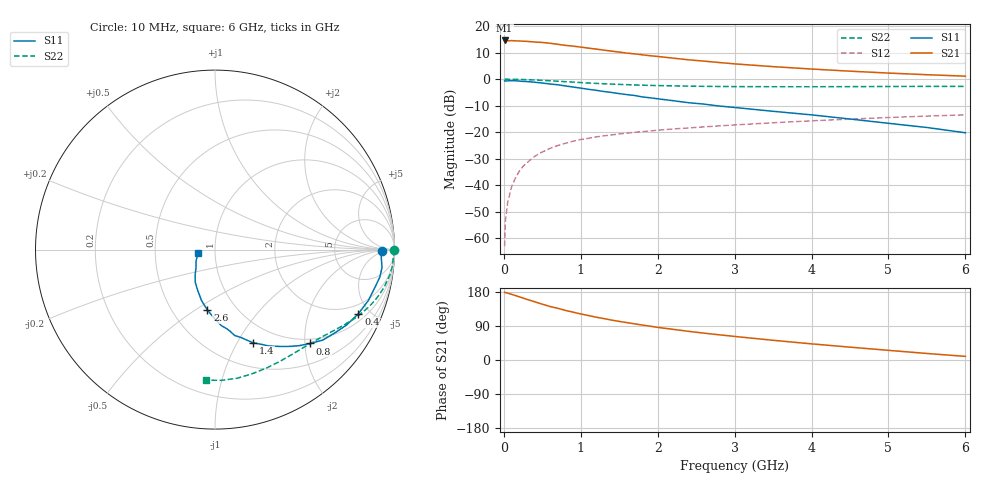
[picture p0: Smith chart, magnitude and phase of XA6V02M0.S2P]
! SIEMENS Discrete & RF Semiconductors
! BFY180
! Si NPN RF Bipolar Junction Transistor in MICRO-X
! VCE = 6 V  IC = 2 mA
! Common Emitter S-Parameters:  May  1997
# GHz  S  MA  R  50
!  f  S11  S21  S12  S22
! GHz  MAG  ANG  MAG  ANG  MAG  ANG  MAG  ANG
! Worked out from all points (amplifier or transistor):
!   36 points, 10 MHz to 6 GHz, reference 50 ohm
!   highest |S21| = 14.6 dB at 10 MHz (marker M1)
!   |S21| within 3 dB of that: start of sweep to 1.127 GHz
!   unconditionally stable (mu >= 1): 3.067 GHz to end of sweep
!   at 250 MHz: K = 0.12, MSG = 23.6 dB, |S12| = -32.9 dB
!   at 1.4 GHz: K = 0.64, MSG = 15.8 dB, |S12| = -21.1 dB
!   at 6 GHz: K = 1.06, MAG = 5.8 dB, |S12| = -13.5 dB
!   S11 on the Smith chart (normalised r, x): 10 MHz: 27, -3; 400 MHz: 1.39, -4.25; 800 MHz: 0.90, -2.12; 1.4 GHz: 0.77, -1.17; 2.6 GHz: 0.74, -0.56; 6 GHz: 0.83, -0.04
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0.01  0.9302 -0.4  5.383 178.7  0.0007 82.9  0.9952 -0.2
0.02  0.9262 -1.1  5.382 178.0  0.0021 99.5  0.9999 -0.6
0.05  0.928 -3.1  5.292 176.5  0.0047 88.1  0.9955 -1.6
0.1  0.936 -6.1  5.353 173.4  0.0092 84.8  0.9933 -3.3
0.25  0.9081 -15.5  5.211 163.6  0.0226 80.6  0.9846 -8.1
0.3  0.9006 -18.3  5.173 160.0  0.0263 78.6  0.9779 -9.6
0.4  0.8751 -24.1  5.03 153.7  0.0348 74.6  0.9654 -12.5
0.5  0.8446 -29.9  4.936 147.3  0.0421 71.2  0.9491 -15.4
0.6  0.8107 -35.2  4.767 141.1  0.0492 68.4  0.9321 -18.0
0.8  0.745 -44.6  4.345 130.9  0.0614 62.9  0.8956 -22.7
1  0.6766 -52.9  4.034 121.5  0.0724 57.8  0.8627 -26.8
1.1  0.643 -57.0  3.853 117.3  0.0764 55.9  0.8462 -28.5
1.4  0.5606 -67.8  3.384 105.4  0.0883 51.3  0.806 -33.6
1.5  0.5339 -70.7  3.246 101.8  0.0922 49.8  0.7957 -35.0
1.8  0.4619 -79.6  2.881 92.2  0.1023 46.7  0.7693 -39.2
2  0.4259 -85.1  2.682 86.1  0.1085 44.7  0.7565 -41.8
2.2  0.392 -89.4  2.495 80.9  0.1146 42.8  0.7475 -44.6
2.6  0.3381 -97.2  2.192 70.9  0.1255 39.9  0.732 -49.5
3.5  0.2472 -112.9  1.724 52.0  0.1501 33.7  0.7197 -60.5
4.5  0.1766 -128.7  1.415 33.9  0.1758 26.7  0.7223 -73.3
5.5  0.1221 -149.5  1.213 17.2  0.2007 19.0  0.7294 -87.0
6  0.0971 -167.5  1.14 9.6  0.2115 14.9  0.7293 -94.0
